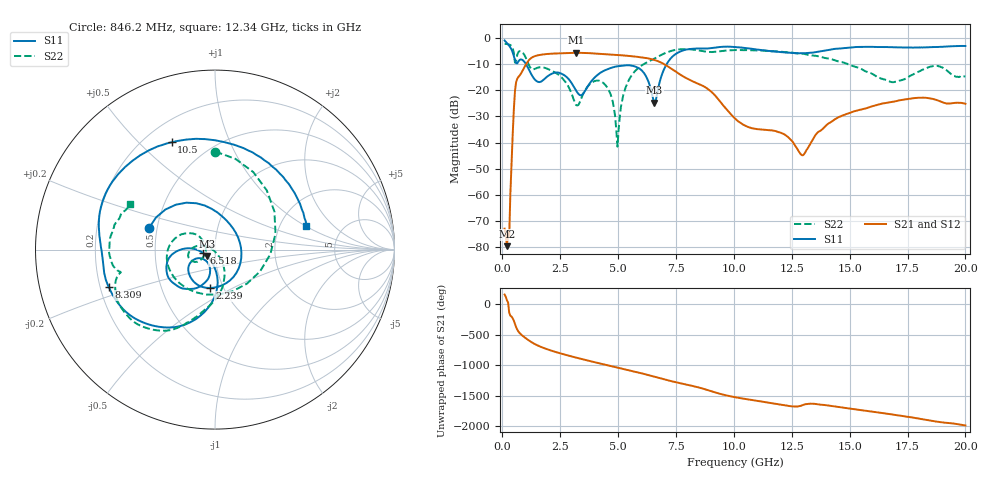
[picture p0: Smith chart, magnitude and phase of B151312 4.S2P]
!  2-Port S-parameters saved by WinCal
! VAR MeasName=S-Parameters (CALIBRATED_DATA) read from VNA (N5244A)
! VAR MeasDate=12/8/2015 5:44:04 PM
! VAR NAME=B151312 4
! VAR FILENAME=B151312 4.S2P
! VAR DATE=12/8/2015 5:44:04 PM
! VAR PHYS_PORTS=1,2
# Hz S DB R 50
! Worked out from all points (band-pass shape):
!   401 points, 100 MHz to 20 GHz, reference 50 ohm
!   highest |S21| = -5.64 dB at 3.184 GHz (marker M1); lowest = -79.6 dB at 199.5 MHz (marker M2)
!   |S21| within 3 dB of the highest: 1.133 GHz to 6.662 GHz (5.529 GHz wide, 142 % of centre)
!   lowest |S11| = -24.7 dB at 6.567 GHz (marker M3), VSWR 1.12, Z = 45.5 - j3.26 ohm
!   |S11| at or under -10 dB: 1.025 GHz to 7.096 GHz (6.071 GHz wide, 150 % of centre)
!   |S22| runs from -41.6 to -2.2 dB; largest |S21 - S12| = 0.0015
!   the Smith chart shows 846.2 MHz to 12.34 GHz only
!   S11 on the Smith chart (normalised r, x): 846.2 MHz: 0.45, +0.13; 2.239 GHz: 0.86, -0.39; 6.518 GHz: 0.88, -0.04; 8.309 GHz: 0.23, -0.16; 10.5 GHz: 0.31, +0.63; 12.34 GHz: 2.81, +1.00
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1e8  -0.91 -41.8  -72.91 156.9  -78.01 167.0  -2.19 169.3
1.995e8  -1.91 -77.0  -79.63 63.8  -76.09 100.5  -2.28 158.2
2.99e8  -2.96 -108.5  -75.71 -141.3  -73.89 169.5  -2.48 145.5
5.4775e8  -8.35 -167.4  -20.27 36.7  -20.27 36.6  -9.40 113.4
8.4625e8  -8.25 161.7  -12.96 -148.7  -12.96 -148.7  -5.25 89.8
1.3935e9  -15.74 59.2  -6.95 69.7  -6.95 69.7  -11.84 -101.8
2.23925e9  -13.31 -98.0  -5.92 -55.2  -5.91 -55.2  -12.99 161.9
3.1845e9  -20.05 -151.5  -5.64 -154.0  -5.64 -154.0  -25.59 167.6
3.43325e9  -21.77 -122.9  -5.66 -178.0  -5.66 -178.0  -22.58 -149.3
4.3785e9  -12.54 -115.3  -6.14 95.6  -6.14 95.6  -17.28 -179.4
4.9755e9  -10.79 -133.7  -6.46 43.1  -6.46 43.1  -41.56 -133.7
5.473e9  -10.40 -150.5  -6.83 -1.3  -6.83 -1.4  -15.98 -70.6
6.51775e9  -23.38 -163.0  -8.24 -100.8  -8.23 -100.8  -8.07 -106.3
6.5675e9  -24.69 -142.2  -8.37 -105.8  -8.36 -105.9  -7.85 -107.3
6.7665e9  -17.92 -86.8  -9.00 -126.5  -9.01 -126.4  -6.92 -112.3
8.30875e9  -4.04 -160.8  -16.91 94.1  -16.89 93.7  -4.49 -158.8
1.005e10  -3.41 132.9  -30.78 -81.7  -30.81 -81.7  -4.58 -177.6
1.049775e10  -3.82 112.0  -33.54 -110.3  -33.62 -110.4  -4.62 175.7
1.23385e10  -5.59 14.3  -37.87 136.5  -37.91 137.0  -5.44 151.8
1.338325e10  -5.58 -29.7  -39.26 172.0  -39.21 172.0  -6.66 138.1
1.67165e10  -3.48 -114.3  -24.59 2.4  -24.41 2.2  -16.57 141.0
2e10  -3.03 -147.4  -25.14 176.4  -25.15 175.3  -14.65 146.0
